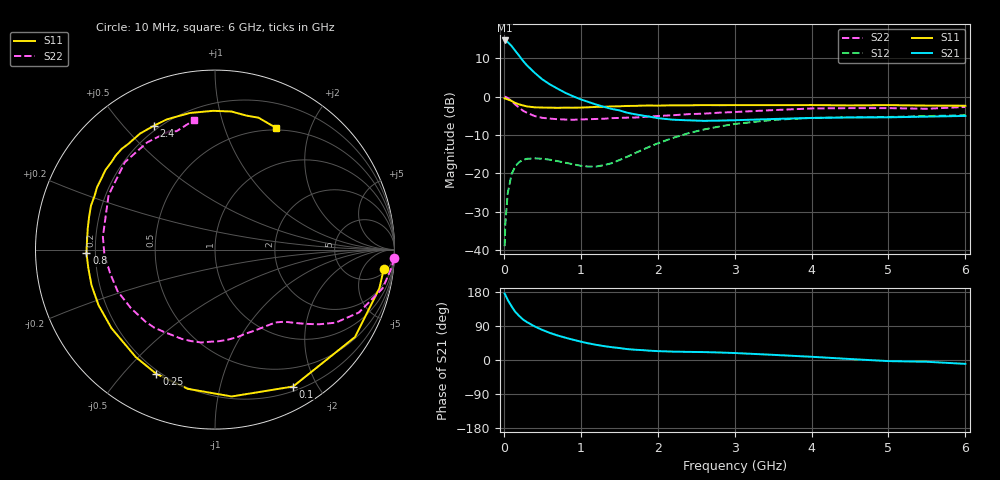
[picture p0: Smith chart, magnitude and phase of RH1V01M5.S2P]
! SIEMENS Small Signal Semiconductors
! BFR106
! Si NPN RF Bipolar Junction Transistor in SOT23
! VCE = 1 V  IC = 1.5 mA
! Common Emitter S-Parameters:  August  1996
# GHz  S  MA  R  50
!  f  S11  S21  S12  S22
! GHz  MAG  ANG  MAG  ANG  MAG  ANG  MAG  ANG
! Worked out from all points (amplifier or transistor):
!   36 points, 10 MHz to 6 GHz, reference 50 ohm
!   highest |S21| = 14.6 dB at 10 MHz (marker M1)
!   |S21| within 3 dB of that: start of sweep to 160.6 MHz
!   unconditionally stable (mu >= 1): 797.6 MHz to end of sweep
!   at 250 MHz: K = 0.31, MSG = 12.9 dB, |S12| = -16.5 dB
!   at 1.4 GHz: K = 1.43, MAG = 3.2 dB, |S12| = -17.4 dB
!   at 6 GHz: K = 1.02, MAG = -1.0 dB, |S12| = -4.9 dB
!   S11 on the Smith chart (normalised r, x): 10 MHz: 7, -14; 100 MHz: 0.25, -1.69; 250 MHz: 0.18, -0.62; 800 MHz: 0.17, -0.01; 2.4 GHz: 0.18, +0.61; 6 GHz: 0.48, +1.52
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0.01  0.9468 -6.5  5.391 175.2  0.0112 86.6  0.9977 -2.8
0.02  0.9409 -13.2  5.387 171.7  0.0222 82.7  0.9914 -5.4
0.05  0.9195 -32.0  5.141 158.8  0.0545 71.8  0.9587 -13.0
0.1  0.8781 -60.3  4.571 141.9  0.097 57.1  0.8751 -23.6
0.15  0.8236 -83.5  3.937 126.7  0.1238 44.4  0.7859 -31.2
0.2  0.7904 -101.1  3.4 116.2  0.14 36.4  0.7133 -35.7
0.25  0.7657 -115.2  2.921 106.8  0.1493 29.9  0.6532 -39.3
0.3  0.744 -126.4  2.555 100.0  0.1543 25.5  0.6147 -41.8
0.4  0.7241 -142.8  2.045 88.7  0.1565 19.0  0.5575 -46.1
0.5  0.719 -154.5  1.676 79.4  0.1544 15.2  0.528 -50.2
0.6  0.7161 -164.0  1.44 71.4  0.1502 13.3  0.5157 -54.7
0.8  0.7163 -178.4  1.119 58.9  0.1373 14.2  0.5015 -64.7
1.1  0.7251 165.2  0.85 43.9  0.1222 25.4  0.5064 -81.2
1.6  0.7545 143.9  0.617 28.9  0.1636 52.6  0.5309 -110.3
2.2  0.7697 122.9  0.499 22.1  0.2895 54.1  0.5709 -145.2
2.4  0.7695 116.3  0.49 21.4  0.3332 50.6  0.5901 -156.8
2.8  0.7712 105.4  0.486 19.8  0.4069 41.9  0.6166 -177.4
3.5  0.7733 90.7  0.51 13.6  0.4964 26.1  0.666 152.9
4.5  0.7668 76.9  0.534 2.6  0.5374 7.8  0.7068 122.3
5  0.7738 71.7  0.536 -2.9  0.5421 1.0  0.7071 111.0
5.5  0.7628 66.9  0.548 -4.7  0.5565 -2.3  0.6935 108.0
6  0.7591 63.2  0.559 -10.2  0.571 -9.0  0.7321 99.0
